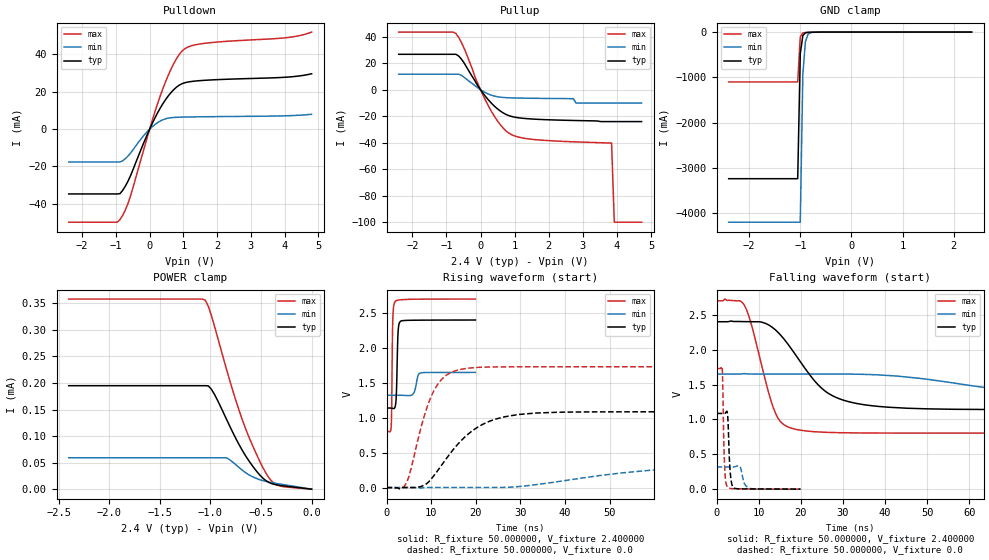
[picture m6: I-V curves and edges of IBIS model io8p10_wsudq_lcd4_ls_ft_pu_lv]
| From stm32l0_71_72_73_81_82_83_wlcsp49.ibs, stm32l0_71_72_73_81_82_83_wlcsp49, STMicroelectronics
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|   Model io8p10_wsudq_lcd4_ls_ft_pu_lv
[Model]  io8p10_wsudq_lcd4_ls_ft_pu_lv
Model_type I/O
Polarity   Non-Inverting
Enable   Active-Low
Vinl =   0.720000V
Vinh =   1.680000V
Vmeas =  1.200000V
Cref =   50.000000pF
Rref =   100.000000M
Vref =   0.0V
C_comp   3.178800pF   3.170000pF   3.206700pF
[Temperature Range]   25.000000   0.105000k   -40.000000
[Pullup Reference]   2.400000V   1.650000V   2.700000V
[Pulldown Reference]   0.0V   0.0V   0.0V
[POWER Clamp Reference]   2.400000V   1.650000V   2.700000V
[GND Clamp Reference]   0.0V   0.0V   0.0V
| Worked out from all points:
|   slope of the pulldown table from 0 to 0.36 V, typ, clamps not added: 28.5 ohm
|   slope of the pullup table from 0 to 0.36 V, typ, clamps not added: 32.2 ohm
|   GND clamp passes 1 mA (typ) near -0.64 V on its own axis
|   rising waveform, R_fixture 50.000000, V_fixture 2.400000: 20-80 % time 296ps typ, 642ps min, 211ps max; typ from 1.14 V to 2.4 V
|   rising waveform, R_fixture 50.000000, V_fixture 0.0: 20-80 % time 9.35ns typ, 24.6ns min, 4.82ns max; typ from 0.001 V to 1.09 V
|   falling waveform, R_fixture 50.000000, V_fixture 2.400000: 20-80 % time 10ns typ, 27.9ns min, 4.94ns max; typ from 2.4 V to 1.14 V
|   falling waveform, R_fixture 50.000000, V_fixture 0.0: 20-80 % time 494ps typ, 852ps min, 396ps max; typ from 1.09 V to 0.001 V
[Pulldown]
|Voltage   I(typ)   I(min)   I(max)
-2.4V     -34.7mA    -17.6mA    -49.82mA
-960mV    -34.7mA    -17.6mA    -49.82mA
-880mV    -34.55mA   -17.6mA    -48.46mA
-720mV    -30.52mA   -15.8mA    -43.27mA
-560mV    -24.65mA   -12.68mA   -35.33mA
0V        0A         0A         0A
400mV     13.84mA    5.066mA    22.03mA
720mV     21.25mA    6.254mA    35.26mA
1.04V     24.83mA    6.464mA    43.02mA
1.6V      26.11mA    6.627mA    45.88mA
4V        27.76mA    7.125mA    48.87mA
4.8V      29.63mA    7.94mA     51.96mA
[Pullup]
|Voltage   I(typ)   I(min)   I(max)
-2.4V     26.83mA    11.83mA    43.61mA
-720mV    26.83mA    11.83mA    42.44mA
-480mV    20.19mA    9.416mA    31.24mA
-160mV    6.617mA    3.074mA    9.467mA
240mV     -7.917mA   -3.299mA   -12.65mA
560mV     -15.67mA   -5.497mA   -25.76mA
880mV     -19.92mA   -6.062mA   -33.51mA
1.68V     -22.29mA   -6.449mA   -37.81mA
2.8V      -23.2mA    -10mA      -39.35mA
3.84V     -24mA      -10mA      -40.2mA
3.92V     -24mA      -10mA      -100mA
4.72V     -24mA      -10mA      -100mA
[GND_clamp]
|Voltage   I(typ)   I(min)   I(max)
-2.4V     -3.238A    -4.199A    -1.101A
-1.05V    -3.238A    -4.199A    -1.101A
-1V       -476.5mA   -4.199A    -104.7mA
-950mV    -76.68mA   -936.1mA   -18.74mA
-900mV    -16.85mA   -213.2mA   -9.358mA
-850mV    -6.706mA   -51.12mA   -6.778mA
-800mV    -4.108mA   -13.92mA   -4.995mA
-650mV    -1.07mA    -1.211mA   -1.175mA
2.35V     0A         0A         0A
[POWER_clamp]
|Voltage   I(typ)   I(min)   I(max)
-2.4V     195uA      59.14uA    358.2uA
-1.05V    195uA      59.14uA    356uA
-1.02V    194.5uA    59.14uA    344.5uA
-960mV    178.7uA    59.14uA    307.4uA
-840mV    131.4uA    59.14uA    225.5uA
-690mV    74.82uA    36.58uA    133.7uA
-600mV    48.08uA    24.92uA    89.53uA
-510mV    26.23uA    17.69uA    51.64uA
-450mV    15.91uA    14.53uA    29.77uA
-390mV    10.19uA    12.23uA    14.39uA
-330mV    7.608uA    10.25uA    6.963uA
0V        0A         0A         0A
[Ramp]
| variable   typ   min   max
dV/dt_r  0.65095/9.34279n   0.19037/24.56799n   1.03799/4.80715n
dV/dt_f  0.75618/10.02980n   0.19644/27.85662n   1.13779/4.93199n
R_load = 50.000000
[Rising Waveform]
R_fixture= 50.000000
V_fixture= 2.400000
V_fixture_min= 1.650000
V_fixture_max= 2.700000
|time   V(typ)   V(min)   V(max)
0s        1.14V      1.323V     803.7mV
1.041ns   1.139V     1.323V     869.3mV
1.161ns   1.138V     1.323V     1.18V
1.401ns   1.135V     1.323V     2.393V
1.882ns   1.15V      1.323V     2.66V
2.202ns   1.336V     1.323V     2.677V
2.603ns   2.241V     1.323V     2.685V
3.043ns   2.376V     1.323V     2.689V
7.648ns   2.398V     1.642V     2.699V
19.94ns   2.4V       1.65V      2.7V
[Rising Waveform]
R_fixture= 50.000000
V_fixture= 0.0
V_fixture_min= 0.0
V_fixture_max= 0.0
|time   V(typ)   V(min)   V(max)
0s        880.2uV    1.329mV    513.6uV
4.505ns   1.735mV    1.425mV    71.25mV
8.509ns   38.97mV    1.537mV    1.037V
11.51ns   248mV      2.317mV    1.483V
18.02ns   751.6mV    2.339mV    1.709V
26.03ns   1.008V     3.76mV     1.729V
38.54ns   1.08V      87.4mV     1.73V
59.06ns   1.086V     248.6mV    1.73V
86.09ns   1.086V     310.1mV    1.73V
249.2ns   1.086V     318.6mV    1.73V
[Falling Waveform]
R_fixture= 50.000000
V_fixture= 2.400000
V_fixture_min= 1.650000
V_fixture_max= 2.700000
|time   V(typ)   V(min)   V(max)
0s        2.4V       1.65V      2.7V
6.507ns   2.402V     1.657V     2.647V
8.008ns   2.401V     1.651V     2.415V
14.01ns   2.281V     1.65V      1.087V
16.52ns   2.112V     1.65V      905.7mV
21.02ns   1.73V      1.65V      836.1mV
29.03ns   1.299V     1.65V      810.1mV
45.55ns   1.16V      1.605V     804mV
91.59ns   1.14V      1.353V     803.7mV
249.2ns   1.14V      1.323V     803.7mV
[Falling Waveform]
R_fixture= 50.000000
V_fixture= 0.0
V_fixture_min= 0.0
V_fixture_max= 0.0
|time   V(typ)   V(min)   V(max)
0s        1.086V     318.6mV    1.73V
1.321ns   1.086V     318.6mV    1.745V
1.441ns   1.086V     318.6mV    1.592V
1.922ns   1.085V     318.6mV    332mV
2.563ns   1.097V     318.6mV    35.62mV
3.203ns   278.3mV    318.4mV    11.96mV
3.924ns   27.3mV     318.3mV    7.624mV
5.485ns   5.153mV    329.6mV    5.245mV
7.928ns   3.747mV    10.83mV    2.55mV
19.94ns   880.2uV    1.329mV    513.6uV
